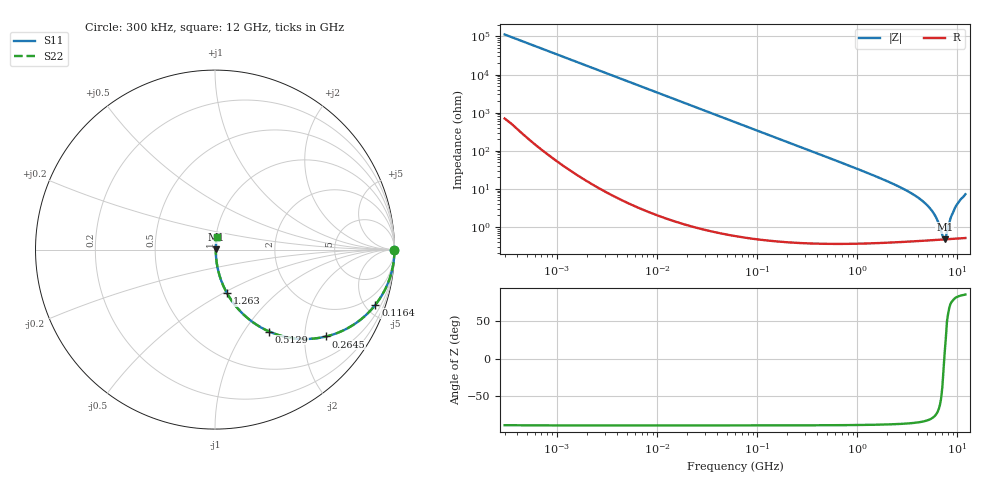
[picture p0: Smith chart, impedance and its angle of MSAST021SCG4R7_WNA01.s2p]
! MSAST021SCG4R7_WNA01  S-PARAMETER MODEL  ( General Type )
! Model Generated by TAIYO YUDEN Corporation (http://www.ty-top.com)
! Version 2.0
! TAIYO YUDEN Control No. 181101
! Copyright(c) 2015 TAIYO YUDEN CO.,LTD. All Rights Reserved.
! Product Description (link to TY-COMPAS)
! https://ds.yuden.co.jp/TYCOMPAS/or/detail?pn=MSAST021SCG4R7BWNA01&u=M
! Products Name : Multilayer Ceramic Capacitors
! Characteristics :
!  Capacitance : 4.7 pF , Rated Voltage : 25V , TCC : CG / C0G
!  Case Size : 0.25 x 0.125 / 0.0098 x 0.0049 [mm/inch] , Thickness : 0.125 / 0.0049 [mm/inch]
!  (Conditions: Temperature = 25 degC , DC Bias Current/Voltage = 0A / 0V)
! External Node Assignments :
!  1  o---| |---o  2
! GND o---------o GND
! Frequency Range : 0.3MHz  -  12000MHz  [ 401 STEP ]
# MHz S RI R 50
! Freq[MHz].  S11 Real  S11 Imag  S21 Real  S21 Imag  S12 Real  S12 Imag  S22 Real  S22 Imag
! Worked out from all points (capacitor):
!   401 points, 300 kHz to 12 GHz, reference 50 ohm
!   read as one part in series: C = 4.7 pF near 316.3 kHz
!   lowest |Z| = 472 mohm at 7.449 GHz (marker M1)
!   series resonance near 7.382 GHz, so ESL is about 99 pH
!   S11 on the Smith chart (normalised r, x): 300 kHz: open; 116.4 MHz: 1.01, -5.82; 264.5 MHz: 1.01, -2.56; 512.9 MHz: 1.01, -1.31; 1.263 GHz: 1.01, -0.52; 12 GHz: 1.01, +0.14
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0.3  1 -0.000886  6.28e-06 0.000886  6.28e-06 0.000886  1 -0.000886
1.769972  1 -0.00523  3.25e-05 0.00523  3.25e-05 0.00523  1 -0.00523
10.44266  0.999 -0.0308  0.000968 0.0308  0.000968 0.0308  0.999 -0.0308
60  0.9694 -0.1717  0.0306 0.1717  0.0306 0.1717  0.9694 -0.1717
116.3536  0.894 -0.3071  0.106 0.3071  0.106 0.3071  0.894 -0.3071
264.5085  0.6201 -0.4839  0.3799 0.4839  0.3799 0.4839  0.6201 -0.4839
353.9943  0.4768 -0.4976  0.5232 0.4976  0.5232 0.4976  0.4768 -0.4976
512.9422  0.3025 -0.4566  0.6975 0.4566  0.6975 0.4566  0.3025 -0.4566
783.7017  0.1564 -0.3591  0.8436 0.3591  0.8436 0.3591  0.1564 -0.3591
1262.535  0.0664 -0.2421  0.9336 0.2421  0.9336 0.2421  0.0664 -0.2421
2088.533  0.0253 -0.1447  0.9747 0.1447  0.9747 0.1447  0.0253 -0.1447
3454.93  0.00983 -0.0753  0.9902 0.0753  0.9902 0.0753  0.00983 -0.0753
4875.354  0.00582 -0.0385  0.9942 0.0385  0.9942 0.0385  0.00582 -0.0385
5868.704  0.0049 -0.0207  0.9951 0.0207  0.9951 0.0207  0.0049 -0.0207
6354.153  0.00471 -0.0133  0.9953 0.0133  0.9953 0.0133  0.00471 -0.0133
7064.448  0.00462 -0.0036  0.9954 0.0036  0.9954 0.0036  0.00462 -0.0036
7448.838  0.00465 0.000611  0.9953 -0.000611  0.9953 -0.000611  0.00465 0.000611
7648.807  0.00468 0.00235  0.9953 -0.00235  0.9953 -0.00235  0.00468 0.00235
8732.115  0.00514 0.019  0.9949 -0.019  0.9949 -0.019  0.00514 0.019
9454.42  0.00581 0.031  0.9942 -0.031  0.9942 -0.031  0.00581 0.031
10511.28  0.00722 0.0477  0.9928 -0.0477  0.9928 -0.0477  0.00722 0.0477
12000  0.0101 0.0705  0.9899 -0.0705  0.9899 -0.0705  0.0101 0.0705
